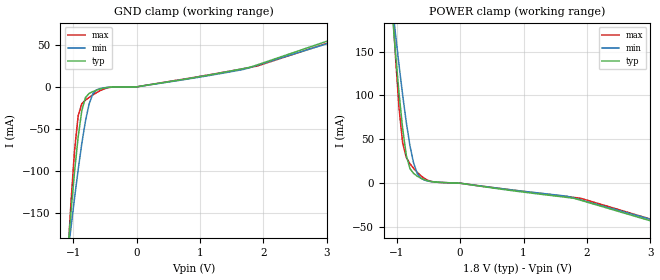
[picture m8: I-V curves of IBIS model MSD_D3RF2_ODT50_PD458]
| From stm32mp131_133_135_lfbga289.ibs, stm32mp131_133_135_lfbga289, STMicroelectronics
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[Model] MSD_D3RF2_ODT50_PD458
Model_type   Input
C_comp 2.281pF   2.243pF   2.310pF
Vinh = 1.150V
Vinl = 650.000mV
[Temperature Range]   25.000   125.000   -40.000
[Voltage Range]   1.800V   1.700V   1.900V
[GND Clamp Reference]   0.00V   0.00V   0.00V
[POWER Clamp Reference]   1.800V   1.700V   1.900V
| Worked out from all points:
|   GND clamp passes 1 mA (typ) near -0.48 V on its own axis
|   POWER clamp passes 1 mA (typ) near -0.31 V on its own axis
[GND Clamp]
-1.785V   -919.5mA   -680.1mA   -1.29A
-1.094V   -204.9mA   -206.3mA   -215mA
-1.036V   -151.2mA   -169.1mA   -139.7mA
-978.8mV  -101.9mA   -133.1mA   -76.77mA
-921.2mV  -59.73mA   -98.92mA   -34.62mA
-863.6mV  -28.42mA   -67.59mA   -20.13mA
-806.1mV  -12.73mA   -40.73mA   -15.79mA
-748.5mV  -7.846mA   -20.38mA   -12.59mA
-690.9mV  -5.634mA   -8.497mA   -9.622mA
-575.8mV  -2.55mA    -1.956mA   -4.54mA
1.785V    23.39mA    22.97mA    23.05mA
3.57V     69.03mA    64.7mA     65.87mA
[Power Clamp]
-1.77V    921mA      689mA      1.287A
-1.079V   202.7mA    209mA      217.6mA
-1.021V   150.3mA    171.4mA    146.4mA
-963.6mV  102.9mA    134.9mA    86.11mA
-906.1mV  62.04mA    100.5mA    45.81mA
-848.5mV  31.65mA    69.22mA    29.1mA
-790.9mV  16.56mA    42.69mA    22.18mA
-733.3mV  11.08mA    22.82mA    16.88mA
-618.2mV  5.642mA    5.703mA    8.424mA
-387.9mV  1.344mA    1.246mA    1.167mA
1.8V      -17.31mA   -17.02mA   -16.28mA
3.585V    -55.38mA   -52.8mA    -53.58mA
